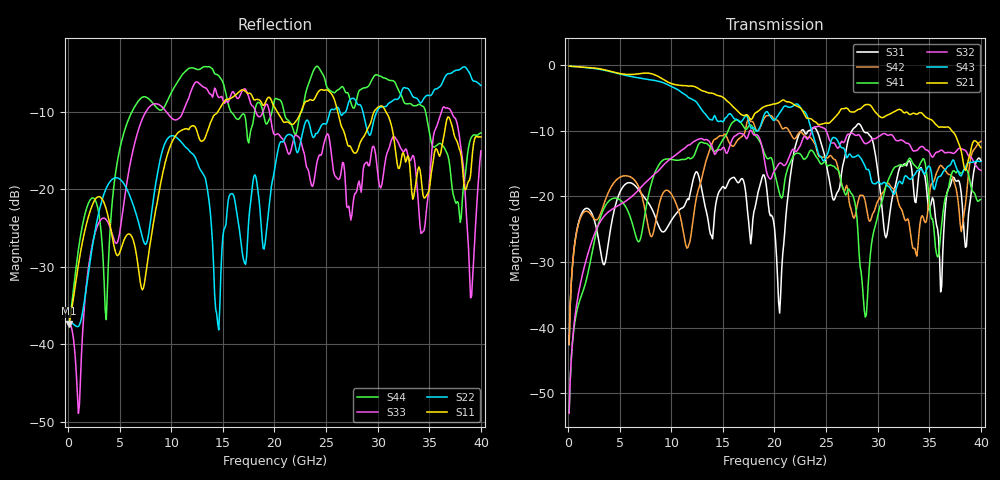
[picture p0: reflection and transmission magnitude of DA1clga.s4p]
! ADC12DJ3200QML-SP
! 196-pin ZMX package
! CLGA Ceramic Package without columns (ceramic land grid array)
! Texas Instruments 4/21/2021
! Single-ended  S-parameters
! PORT#  PORT_NAME  NET_NAME
! PORT1:  DAxN.DIEBUMP DAxN
! PORT2:  DAxN.BGA  DAxN
! PORT3:  DAxP.DIEBUMP DAxP
! PORT4:  DAxP.BGA  DAxP
! Touchstone Ver. 1.0
! Number of ports is 4
# Hz	S	MA	R	50.000000
! SCATTERING PARAMETERS  :
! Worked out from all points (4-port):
!   400 points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, 100 MHz to 40 GHz, reference 50 ohm
!   strongest paths, dB at 100 MHz, 10.1 GHz, 20.1 GHz, 30.1 GHz, 40 GHz:
!     S21: -0.1, -2.8, -5.9, -7.7, -12.6
!     S43: -0.1, -3.3, -8.2, -17.8, -14.6
!     S32: -53.1, -14.0, -15.8, -10.8, -16.0
!     S41: -53.0, -14.4, -17.0, -22.2, -20.5
!     S42: -42.6, -19.9, -8.3, -20.5, -11.6
!     S31: -42.6, -23.4, -26.6, -17.2, -14.6
!   lowest |S11| = -37.4 dB at 100 MHz (marker M1), VSWR 1.03, Z = 51.4 - j0.106 ohm
!   |S11| at or under -10 dB: start of sweep to 14.51 GHz; 26.13 GHz to 29.65 GHz (3.521 GHz wide, 12.6 % of centre); 30.8 GHz to end of sweep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
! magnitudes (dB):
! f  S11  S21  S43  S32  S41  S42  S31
! 100 MHz  -37.4  -0.1  -0.1  -53.1  -53.0  -42.6  -42.6
! 3.6 GHz  -22.2  -0.7  -0.8  -22.8  -21.4  -20.6  -30.0
! 16.2 GHz  -7.9  -6.6  -8.2  -10.8  -8.4  -11.9  -17.3
! 20.5 GHz  -10.5  -5.6  -7.3  -14.9  -19.6  -8.8  -37.8
! 28.8 GHz  -12.8  -6.0  -15.5  -11.9  -38.4  -20.8  -10.3
! 36.1 GHz  -15.4  -9.4  -16.9  -12.9  -25.7  -15.3  -34.6
! 40 GHz  -13.3  -12.6  -14.6  -16.0  -20.5  -11.6  -14.6
